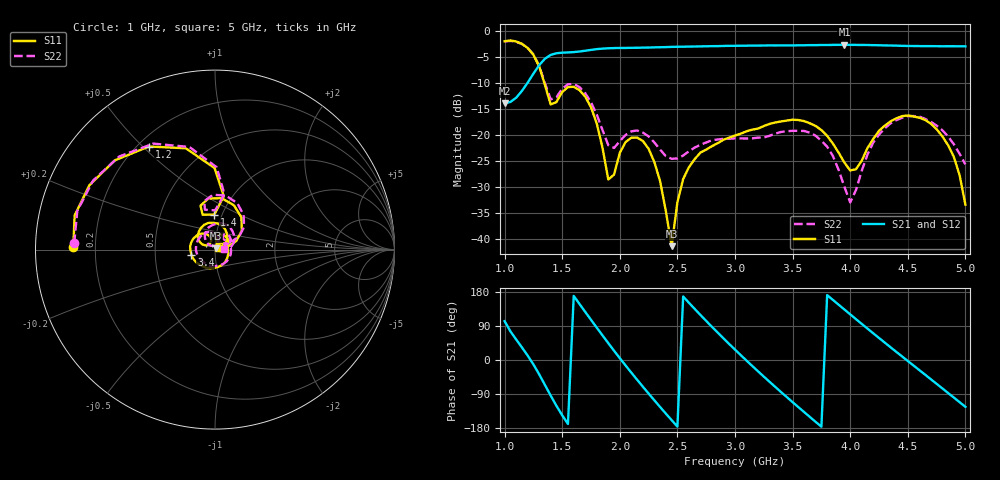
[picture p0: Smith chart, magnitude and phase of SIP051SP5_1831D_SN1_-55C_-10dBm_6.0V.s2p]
# GHz  S  dB  R  50
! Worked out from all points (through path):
!   81 points, 1 GHz to 5 GHz, reference 50 ohm
!   highest |S21| = -2.72 dB at 3.95 GHz (marker M1); lowest = -13.9 dB at 1 GHz (marker M2)
!   lowest |S11| = -41.4 dB at 2.45 GHz (marker M3), VSWR 1.02, Z = 50.6 + j0.626 ohm
!   |S11| at or under -10 dB: 1.344 GHz to end of sweep
!   |S22| runs from -33.0 to -2.0 dB; largest |S21 - S12| = 0.0023
!   S11 on the Smith chart (normalised r, x): 1 GHz: 0.12, +0.01; 1.2 GHz: 0.24, +0.52; 1.4 GHz: 0.92, +0.37; 3.4 GHz: 0.77, -0.05; 5 GHz: 1.04, +0.02
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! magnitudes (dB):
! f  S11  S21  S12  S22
! 1 GHz  -2.0  -13.9  -13.9  -2.1
! 1.2 GHz  -3.3  -10.0  -10.0  -3.3
! 1.4 GHz  -14.2  -4.7  -4.7  -13.2
! 1.55 GHz  -10.8  -4.2  -4.2  -10.3
! 1.7 GHz  -12.7  -3.9  -3.9  -12.0
! 1.8 GHz  -17.8  -3.6  -3.6  -16.1
! 1.9 GHz  -28.6  -3.4  -3.4  -22.0
! 2.15 GHz  -20.5  -3.3  -3.3  -19.2
! 2.35 GHz  -28.9  -3.2  -3.2  -22.8
! 2.45 GHz  -41.4  -3.1  -3.1  -24.6
! 2.5 GHz  -32.9  -3.1  -3.1  -24.5
! 2.6 GHz  -26.2  -3.1  -3.1  -23.2
! 3 GHz  -20.1  -2.9  -2.9  -20.7
! 3.4 GHz  -17.4  -2.8  -2.8  -19.4
! 3.7 GHz  -18.3  -2.8  -2.8  -20.2
! 3.95 GHz  -25.3  -2.7  -2.7  -30.0
! 4 GHz  -26.8  -2.7  -2.7  -33.0
! 4.2 GHz  -20.8  -2.8  -2.8  -21.5
! 4.35 GHz  -17.4  -2.9  -2.9  -17.8
! 4.75 GHz  -18.9  -3.0  -3.0  -18.2
! 4.9 GHz  -24.3  -3.0  -3.0  -21.8
! 5 GHz  -33.4  -3.0  -3.0  -25.7
